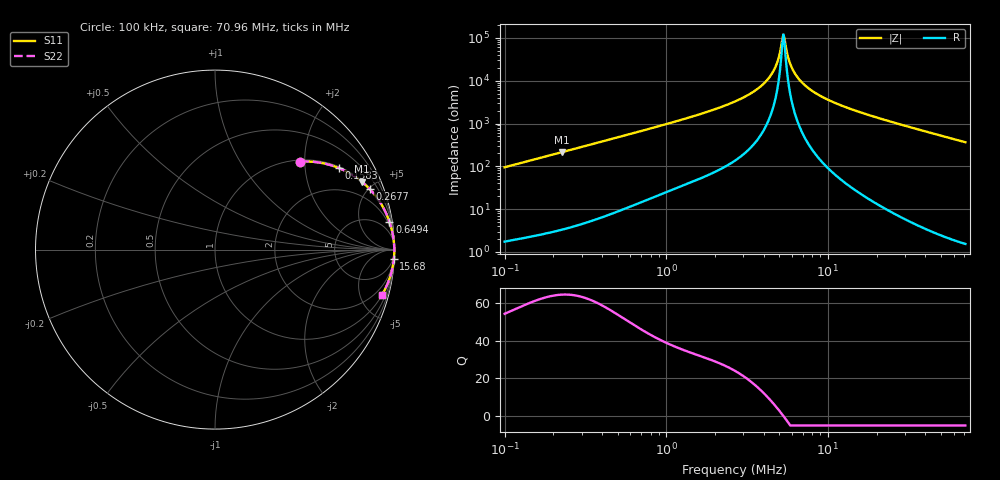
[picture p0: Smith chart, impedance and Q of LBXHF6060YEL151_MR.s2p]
! LBXHF6060YEL151_MR  S-PARAMETER MODEL  ( General Type )
! Model Generated by TAIYO YUDEN Corporation (http://www.ty-top.com)
! Version 1.0
! TAIYO YUDEN Control No. 200217NI43SB-FBB
! Copyright(c) 2020 TAIYO YUDEN CO.,LTD. All Rights Reserved.
! Product Description (link to TY-COMPAS)
! https://ds.yuden.co.jp/TYCOMPAS/or/detail?pn=LBXHF6060YEL151MMR&u=M
! Products Name : Inductors
! Characteristics :
!  Inductance : 150 uH , SRF(min) : 3.5 MHz , DC Resistance(max) : 0.816 Ohm
!  Rated Current : Saturation :830 mA , Temp Rise : 480 mA
!  Case Size : 6.0 x 6.0 / 0.236 x 0.236 [mm/inch] , Thickness : 4.5 / 0.177 [mm/inch]
!  (Conditions: Temperature = 25 degC , DC Bias Current/Voltage = 0A / 0V)
! External Node Assignments :
!  1  o---GGG---o  2
! GND o---------o GND
! Frequency Range : 0.1MHz  -  70.9631MHz  [ 402 STEP ]
# MHz S RI R 50
! Freq[MHz].  S11 Real  S11 Imag  S21 Real  S21 Imag  S12 Real  S12 Imag  S22 Real  S22 Imag
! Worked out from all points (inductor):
!   401 points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, 100 kHz to 70.96 MHz, reference 50 ohm
!   read as one part in series: L = 151 uH near 103.3 kHz
!   highest Q = 64.6 at 227.2 kHz (marker M1), where L = 151 uH
!   self-resonance near 5.307 MHz
!   S11 on the Smith chart (normalised r, x): 100 kHz: 1.03, +1.90; 158.3 kHz: 1.05, +3.00; 267.7 kHz: 1.08, +5.07; 649.4 kHz: 1, +12; 15.68 MHz: 1, -37; 70.96 MHz: 1.03, -7.30
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0.1  0.4749 0.4903  0.5251 -0.4903  0.5251 -0.4903  0.4749 0.4903
0.158333  0.6895 0.4547  0.3105 -0.4547  0.3105 -0.4547  0.6895 0.4547
0.227185  0.8184 0.3779  0.1816 -0.3779  0.1816 -0.3779  0.8184 0.3779
0.267704  0.8613 0.3379  0.1387 -0.3379  0.1387 -0.3379  0.8613 0.3379
0.300295  0.886 0.31  0.114 -0.31  0.114 -0.31  0.886 0.31
0.649448  0.9714 0.1565  0.0286 -0.1565  0.0286 -0.1565  0.9714 0.1565
0.90177  0.9842 0.1131  0.0158 -0.1131  0.0158 -0.1131  0.9842 0.1131
2.70797  0.9979 0.0296  0.00213 -0.0296  0.00213 -0.0296  0.9979 0.0296
3.579421  0.9987 0.0166  0.0013 -0.0166  0.0013 -0.0166  0.9987 0.0166
4.287619  0.999 0.00886  0.001 -0.00886  0.001 -0.00886  0.999 0.00886
4.809603  0.9991 0.00409  0.000887 -0.00409  0.000887 -0.00409  0.9991 0.00409
5.135935  0.9992 0.00139  0.000846 -0.00139  0.000846 -0.00139  0.9992 0.00139
5.307313  0.9992 4.05e-05  0.000833 -4.05e-05  0.000833 -4.05e-05  0.9992 4.05e-05
5.484409  0.9992 -0.00131  0.000823 0.00131  0.000823 0.00131  0.9992 -0.00131
5.856528  0.9992 -0.00401  0.000817 0.00401  0.000817 0.00401  0.9992 -0.00401
6.253894  0.9992 -0.00674  0.000829 0.00674  0.000829 0.00674  0.9992 -0.00674
6.901063  0.9991 -0.0109  0.000879 0.0109  0.000879 0.0109  0.9991 -0.0109
7.999526  0.999 -0.0173  0.00103 0.0173  0.00103 0.0173  0.999 -0.0173
10.57385  0.9984 -0.0306  0.00164 0.0306  0.00164 0.0306  0.9984 -0.0306
15.67816  0.9964 -0.0536  0.00357 0.0536  0.00357 0.0536  0.9964 -0.0536
24.02217  0.9915 -0.0879  0.00849 0.0879  0.00849 0.0879  0.9915 -0.0879
70.9631  0.9293 -0.2542  0.0707 0.2542  0.0707 0.2542  0.9293 -0.2542
